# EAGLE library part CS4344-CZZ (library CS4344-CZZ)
Audio D/A Converter ICs Stereo DAC 24-Bit 192kHz Source: Datasheet
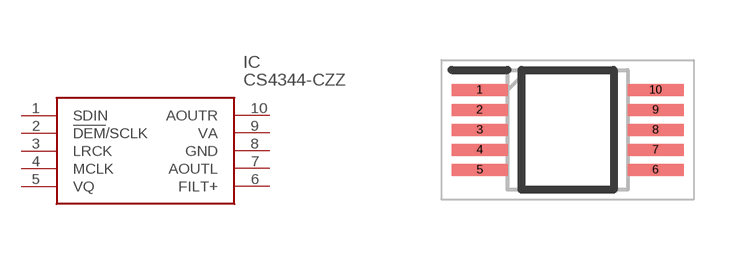
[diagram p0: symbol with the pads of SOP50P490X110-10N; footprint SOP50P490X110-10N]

Designator prefix IC

## CS4344-CZZ (Description: Audio D/A Converter ICs Stereo DAC 24-Bit 192kHz; Height: 1.1mm; Manufacturer_Name: Cirrus Logic; Manufacturer_Part_Number: CS4344-CZZ; RS_Part_Number: 4915754)  [SOP50P490X110-10N]
1  SDIN
2  !DEM!/SCLK
3  LRCK
4  MCLK
5  VQ
6  FILT+
7  AOUTL
8  GND
9  VA
10  AOUTR

## Footprint SOP50P490X110-10N (pad centres in mm)
CS4344-CZZ
smd 1.4 x 0.3: 1 -2.2,1; 2 -2.2,0.5; 3 -2.2,0; 4 -2.2,-0.5; 5 -2.2,-1; 6 2.2,-1; 7 2.2,-0.5; 8 2.2,0; 9 2.2,0.5; 10 2.2,1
